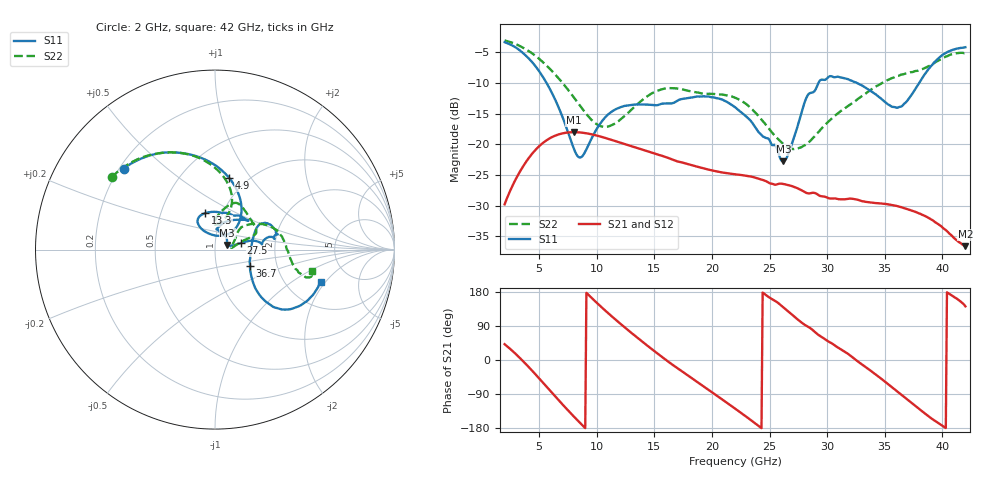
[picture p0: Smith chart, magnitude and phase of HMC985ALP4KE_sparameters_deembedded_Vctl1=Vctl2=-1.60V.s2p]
!s2p File: Measurements: S11, S21, S12, S22
# GHz S dB R 50.0
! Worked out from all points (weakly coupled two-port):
!   401 points, 2 GHz to 42 GHz, reference 50 ohm
!   highest |S21| = -18.02 dB at 8 GHz (marker M1); lowest = -36.6 dB at 42 GHz (marker M2)
!   lowest |S11| = -22.8 dB at 26.2 GHz (marker M3), VSWR 1.16, Z = 57.2 + j2.92 ohm
!   |S11| at or under -10 dB: 5.642 GHz to 29.25 GHz (23.6 GHz wide, 135 % of centre); 32.6 GHz to 37.98 GHz (5.384 GHz wide, 15.3 % of centre)
!   |S22| runs from -20.8 to -3.1 dB; largest |S21 - S12| = 0.00013
!   S11 on the Smith chart (normalised r, x): 2 GHz: 0.22, +0.36; 4.9 GHz: 0.83, +0.79; 13.3 GHz: 0.83, +0.35; 27.5 GHz: 1.33, +0.10; 36.7 GHz: 1.46, -0.27; 42 GHz: 3.09, -1.82
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2  -3.34 138.4  -29.80 41.7  -29.80 41.7  -3.06 145.0
3.4  -4.80 110.3  -24.23 3.1  -24.24 3.1  -4.04 121.8
4.9  -7.82 78.7  -20.48 -45.2  -20.49 -45.2  -5.90 98.0
6.2  -11.97 54.4  -18.75 -89.5  -18.76 -89.5  -8.22 80.6
8  -20.66 58.7  -18.02 -148.8  -18.03 -148.9  -12.32 69.1
8.7  -22.03 91.5  -18.10 -170.6  -18.10 -170.6  -14.10 70.7
10.7  -15.67 123.6  -18.94 131.4  -18.95 131.4  -17.17 89.0
13.3  -13.52 104.9  -20.46 64.4  -20.47 64.4  -13.83 82.9
15.4  -13.55 77.5  -21.74 14.3  -21.74 14.3  -11.17 69.0
18.9  -12.22 42.0  -23.75 -61.8  -23.75 -61.8  -11.61 43.0
22  -13.95 55.7  -24.89 -128.0  -24.90 -128.0  -12.39 20.8
24.5  -18.80 85.6  -25.88 175.7  -25.89 175.6  -16.40 16.1
26.2  -22.79 20.5  -26.48 138.7  -26.48 138.7  -19.97 7.3
27.5  -16.62 14.2  -27.26 105.5  -27.26 105.6  -20.65 8.1
28.7  -11.56 6.7  -27.93 80.3  -27.93 80.3  -19.11 20.7
29.5  -9.46 10.5  -28.48 61.5  -28.49 61.5  -17.45 30.4
31.1  -9.06 18.6  -28.98 30.1  -28.97 30.1  -14.70 40.0
33.3  -10.72 29.5  -29.37 -17.7  -29.38 -17.7  -11.79 33.7
35.4  -13.61 9.2  -29.84 -66.3  -29.84 -66.4  -9.41 21.8
36.7  -13.36 -24.4  -30.43 -97.8  -30.43 -97.9  -8.53 12.5
39.6  -6.10 -42.1  -32.98 -165.4  -32.99 -165.7  -6.41 -14.8
42  -4.16 -17.1  -36.62 141.5  -36.65 141.4  -5.12 -12.2
